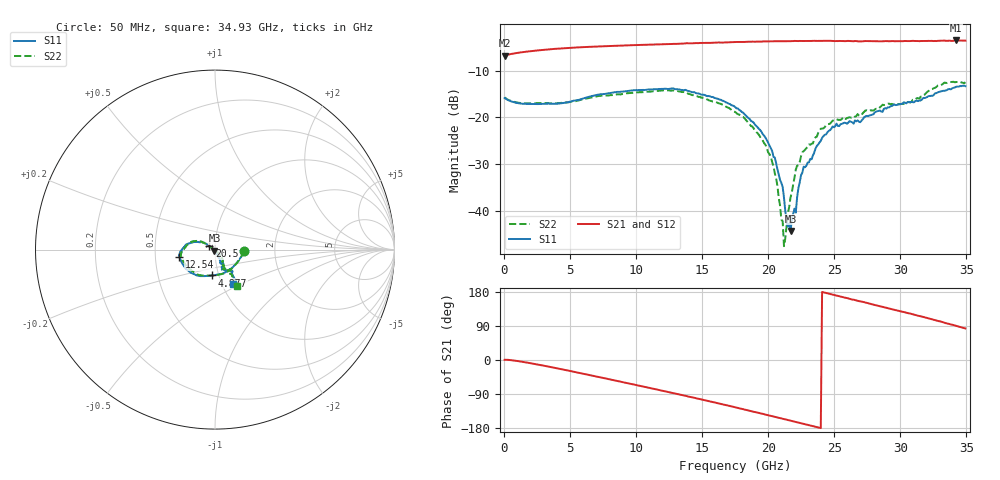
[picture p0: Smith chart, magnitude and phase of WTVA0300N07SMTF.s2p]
! 50 ohm 2-Port S-parameters measured by Modelithics Inc support@modelithics.com  Tampa, FL USA 813-866-6335 (February 2024)
! Smiths Interconnect,  3dB P/N: WTVA0300N07SMTF, Temperature: -50 C
! Board: 10 mil Rogers 4350B, Mounting Pad Dimensions: Length: 15 mils, Width: 25 mils, Gap: 40 mils.
# Hz S RI R 50
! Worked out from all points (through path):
!   352 points, 50 MHz to 34.93 GHz, reference 50 ohm
!   highest |S21| = -3.58 dB at 34.23 GHz (marker M1); lowest = -6.8 dB at 50 MHz (marker M2)
!   group delay of S21, straight-line fit = 22.4 ps
!   lowest |S11| = -44.3 dB at 21.69 GHz (marker M3), VSWR 1.01, Z = 49.7 - j0.533 ohm
!   |S11| at or under -10 dB: start of sweep to end of sweep
!   |S22| runs from -47.5 to -12.4 dB; largest |S21 - S12| = 0.0041
!   S11 on the Smith chart (normalised r, x): 50 MHz: 1.38, -0.02; 4.877 GHz: 0.93, -0.27; 12.54 GHz: 0.67, -0.06; 20.5 GHz: 0.94, +0.04; 34.93 GHz: 1.12, -0.45
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5e7  0.1599 -0.00745  0.4557 0.00357  0.4555 0.00328  0.1634 -0.00743
4.8765e9  -0.0173 -0.144  0.4864 -0.2598  0.486 -0.2597  -0.0135 -0.1441
5.8715e9  -0.0539 -0.1475  0.4576 -0.3245  0.4573 -0.3244  -0.0521 -0.1455
1.1742e10  -0.1926 -0.0574  0.1131 -0.5909  0.1123 -0.5908  -0.185 -0.0517
1.2538e10  -0.1979 -0.0397  0.0504 -0.6043  0.0498 -0.6041  -0.1911 -0.0322
1.7513e10  -0.1214 0.0418  -0.3657 -0.5234  -0.366 -0.523  -0.1029 0.0488
1.98015e10  -0.0509 0.0324  -0.5245 -0.3791  -0.524 -0.3796  -0.0425 0.0275
2.0498e10  -0.0316 0.0197  -0.5623 -0.3256  -0.5625 -0.3248  -0.0222 0.012
2.09955e10  -0.0172 0.0102  -0.5849 -0.2832  -0.5849 -0.2826  -0.00807 0.00013
2.1095e10  -0.0154 0.00927  -0.5895 -0.274  -0.5895 -0.2736  -0.00769 -0.00124
2.11945e10  -0.0121 0.00691  -0.5927 -0.2664  -0.5926 -0.266  -0.00352 -0.0023
2.13935e10  -0.00757 -0.000408  -0.601 -0.2484  -0.601 -0.2478  0.00131 -0.00688
2.1692e10  -0.00289 -0.00536  -0.6113 -0.2243  -0.6112 -0.224  0.00634 -0.0125
2.19905e10  0.00173 -0.0104  -0.6245 -0.1973  -0.6243 -0.1968  0.0165 -0.0157
2.209e10  0.00435 -0.00856  -0.6272 -0.1864  -0.6271 -0.1859  0.0197 -0.0195
2.2488e10  0.0131 -0.0203  -0.6362 -0.1486  -0.6361 -0.1479  0.0262 -0.0283
2.33835e10  0.0186 -0.0344  -0.6524 -0.0645  -0.6521 -0.0641  0.0334 -0.0405
2.39805e10  0.0251 -0.05  -0.6554 -0.00436  -0.6552 -0.00449  0.0435 -0.0618
2.51745e10  0.0352 -0.0781  -0.6436 0.1132  -0.6433 0.1132  0.0458 -0.0839
2.91545e10  0.0566 -0.1145  -0.465 0.4533  -0.4643 0.4535  0.0704 -0.1212
3.4229e10  0.112 -0.1806  -0.00212 0.6624  0.00195 0.6622  0.1303 -0.1996
3.49255e10  0.0984 -0.1917  0.0774 0.6553  0.08 0.6547  0.1228 -0.2032
